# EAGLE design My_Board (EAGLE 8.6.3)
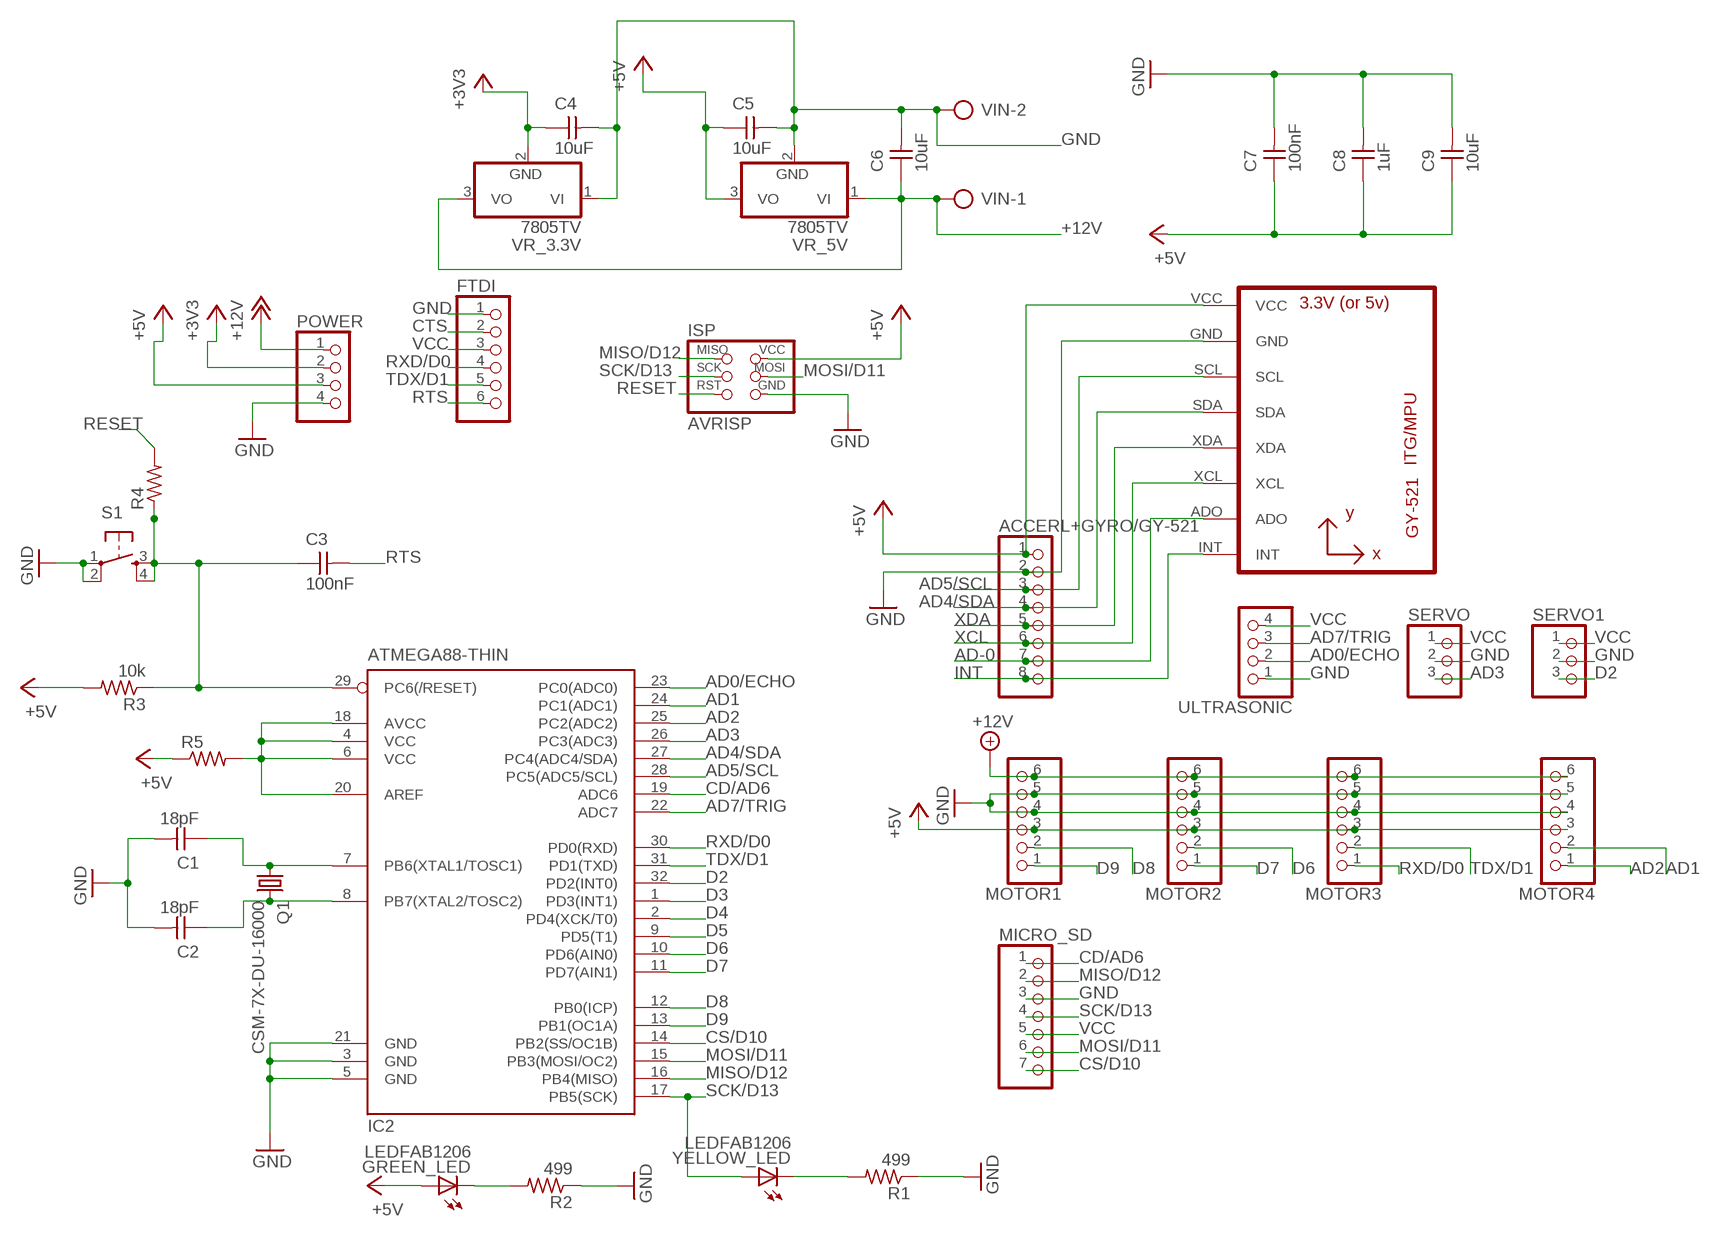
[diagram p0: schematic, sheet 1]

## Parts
ACCERL+GYRO/GY-521  PINHD-1X8  [1X08]
C1  18pF  CAP-UNPOLARIZED  [C1206]
C2  18pF  CAP-UNPOLARIZED  [C1206]
C3  100nF  CAP-UNPOLARIZEDFAB  [C1206FAB]
C4  10uF  CAP-UNPOLARIZEDFAB  [C1206FAB]
C5  10uF  CAP-UNPOLARIZEDFAB  [C1206FAB]
C6  10uF  CAP-UNPOLARIZEDFAB  [C1206FAB]
C7  100nF  CAP-UNPOLARIZEDFAB  [C1206FAB]
C8  1uF  CAP-UNPOLARIZEDFAB  [C1206FAB]
C9  10uF  CAP-UNPOLARIZEDFAB  [C1206FAB]
FTDI  PINHD-1X6  [1X06]
GREEN_LED  LEDFAB1206  [LED1206FAB]
IC2  ATMEGA88-THIN  [TQFP32-08THIN]
ISP  AVRISP  [2X03]
MICRO_SD  PINHD-1X7  [1X07]
MOTOR1  PINHD-1X6  [1X06]
MOTOR2  PINHD-1X6  [1X06]
MOTOR3  PINHD-1X6  [1X06]
MOTOR4  PINHD-1X6  [1X06]
POWER  PINHD-1X4  [1X04]
Q1  CSM-7X-DU-16000  CSM-7X-DU  [CSM-7X-DU]
R1  499  RES-US1206FAB  [R1206FAB]
R2  499  RES-US1206FAB  [R1206FAB]
R3  10k  RES-US1206FAB  [R1206FAB]
R4  RES-US1206FAB  [R1206FAB]
R5  RES-US1206FAB  [R1206FAB]
S1  6MM_SWITCH6MM_SWITCH  [6MM_SWITCH]
SERVO  PINHD-1X3  [1X03]
SERVO1  PINHD-1X3  [1X03]
U1  GY-521MPU6050  [GY-521]
ULTRASONIC  PINHD-1X4  [1X04]
VIN  AK500/2  [AK500/2]
VR_3.3V  7805TV  [TO220V]
VR_5V  7805TV  [TO220V]
YELLOW_LED  LEDFAB1206  [LED1206FAB]

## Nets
+3V3: C4.1 POWER.2 VR_3.3V.2(GND)
+12V: C6.1 MOTOR1.6 MOTOR2.6 MOTOR3.6 MOTOR4.6 POWER.1 VIN.1 VR_3.3V.3(VO) VR_5V.1(VI)
AD0/ECHO: IC2.23(PC0(ADC0)) ULTRASONIC.2
AD1: IC2.24(PC1(ADC1)) MOTOR4.2
AD2: IC2.25(PC2(ADC2)) MOTOR4.1
AD3: IC2.26(PC3(ADC3)) SERVO.3
AD4/SDA: ACCERL+GYRO/GY-521.4 IC2.27(PC4(ADC4/SDA)) U1.SDA
AD5/SCL: ACCERL+GYRO/GY-521.3 IC2.28(PC5(ADC5/SCL)) U1.SCL
AD7/TRIG: IC2.22(ADC7) ULTRASONIC.3
AD-0: ACCERL+GYRO/GY-521.7 U1.ADO
CD/AD6: IC2.19(ADC6) MICRO_SD.1
CS/D10: IC2.14(PB2(SS/OC1B)) MICRO_SD.7
CTS: FTDI.2
D2: IC2.32(PD2(INT0)) SERVO1.3
D3: IC2.1(PD3(INT1))
D4: IC2.2(PD4(XCK/T0))
D5: IC2.9(PD5(T1))
D6: IC2.10(PD6(AIN0)) MOTOR2.2
D7: IC2.11(PD7(AIN1)) MOTOR2.1
D8: IC2.12(PB0(ICP)) MOTOR1.2
D9: IC2.13(PB1(OC1A)) MOTOR1.1
GND: ACCERL+GYRO/GY-521.2 C1.2 C2.2 C4.2 C5.2 C6.2 C7.2 C8.2 C9.2 FTDI.1 IC2.3(GND) IC2.5(GND) IC2.21(GND) ISP.6(GND) MICRO_SD.3 MOTOR1.4 MOTOR1.5 MOTOR2.4 MOTOR2.5 MOTOR3.4 MOTOR3.5 MOTOR4.4 MOTOR4.5 POWER.4 R1.1 R2.1 S1.1(P) S1.2(P1) SERVO1.2 SERVO.2 U1.GND ULTRASONIC.1 VIN.2 VR_3.3V.1(VI) VR_5V.2(GND)
INT: ACCERL+GYRO/GY-521.8 U1.INT
MISO/D12: IC2.16(PB4(MISO)) ISP.1(MISO) MICRO_SD.2
MOSI/D11: IC2.15(PB3(MOSI/OC2)) ISP.4(MOSI) MICRO_SD.6
N$3: R1.2 YELLOW_LED.2(C)
N$5: C2.1 IC2.8(PB7(XTAL2/TOSC2)) Q1.2
N$6: C1.1 IC2.7(PB6(XTAL1/TOSC1)) Q1.1
N$34: GREEN_LED.2(C) R2.2
RESET: C3.1 IC2.29(PC6(/RESET)) ISP.5(RST) R3.1 R4.1 R4.2 S1.3(S) S1.4(S1)
RTS: C3.2 FTDI.6
RXD/D0: FTDI.4 IC2.30(PD0(RXD)) MOTOR3.1
SCK/D13: IC2.17(PB5(SCK)) ISP.3(SCK) MICRO_SD.4 YELLOW_LED.1(A)
TDX/D1: FTDI.5 IC2.31(PD1(TXD)) MOTOR3.2
VCC: ACCERL+GYRO/GY-521.1 C5.1 C7.1 C8.1 C9.1 FTDI.3 GREEN_LED.1(A) IC2.4(VCC) IC2.6(VCC) IC2.18(AVCC) IC2.20(AREF) ISP.2(VCC) MICRO_SD.5 MOTOR1.3 MOTOR2.3 MOTOR3.3 MOTOR4.3 POWER.3 R3.2 R5.1 R5.2 SERVO1.1 SERVO.1 U1.VCC ULTRASONIC.4 VR_5V.3(VO) ; supply symbol labelled +5V
XCL: ACCERL+GYRO/GY-521.6 U1.XCL
XDA: ACCERL+GYRO/GY-521.5 U1.XDA

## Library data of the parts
ACCERL+GYRO/GY-521 = pinhead:PINHD-1X8: PIN HEADER
C1-C9 = fab:CAP-UNPOLARIZED
FTDI MOTOR1-MOTOR4 = pinhead:PINHD-1X6: PIN HEADER
GREEN_LED YELLOW_LED = fab:LED: LED
IC2 = fab:ATMEGA88-THIN
ISP = fab:AVRISP
MICRO_SD = pinhead:PINHD-1X7: PIN HEADER
POWER ULTRASONIC = pinhead:PINHD-1X4: PIN HEADER
Q1 = crystal:CSM-7X-DU: SMD CRYSTAL; OC_FARNELL: unknown; OC_NEWARK: unknown
R1-R5 = fab:RES-US: Resistor (US Symbol)
S1 = fab:6MM_SWITCH: OMRON SWITCH
SERVO SERVO1 = pinhead:PINHD-1X3: PIN HEADER
U1 = gy-521:GY-521
VIN = con-ptr500:AK500/2: CONNECTOR; OC_FARNELL: unknown; OC_NEWARK: unknown
VR_3.3V VR_5V = linear:78*: Positive VOLTAGE REGULATOR Source: http://cache.national.com/ds/LM/LM78L05.pdf http://www.fairchildsemi.com/ds/LM/LM7805.pdf

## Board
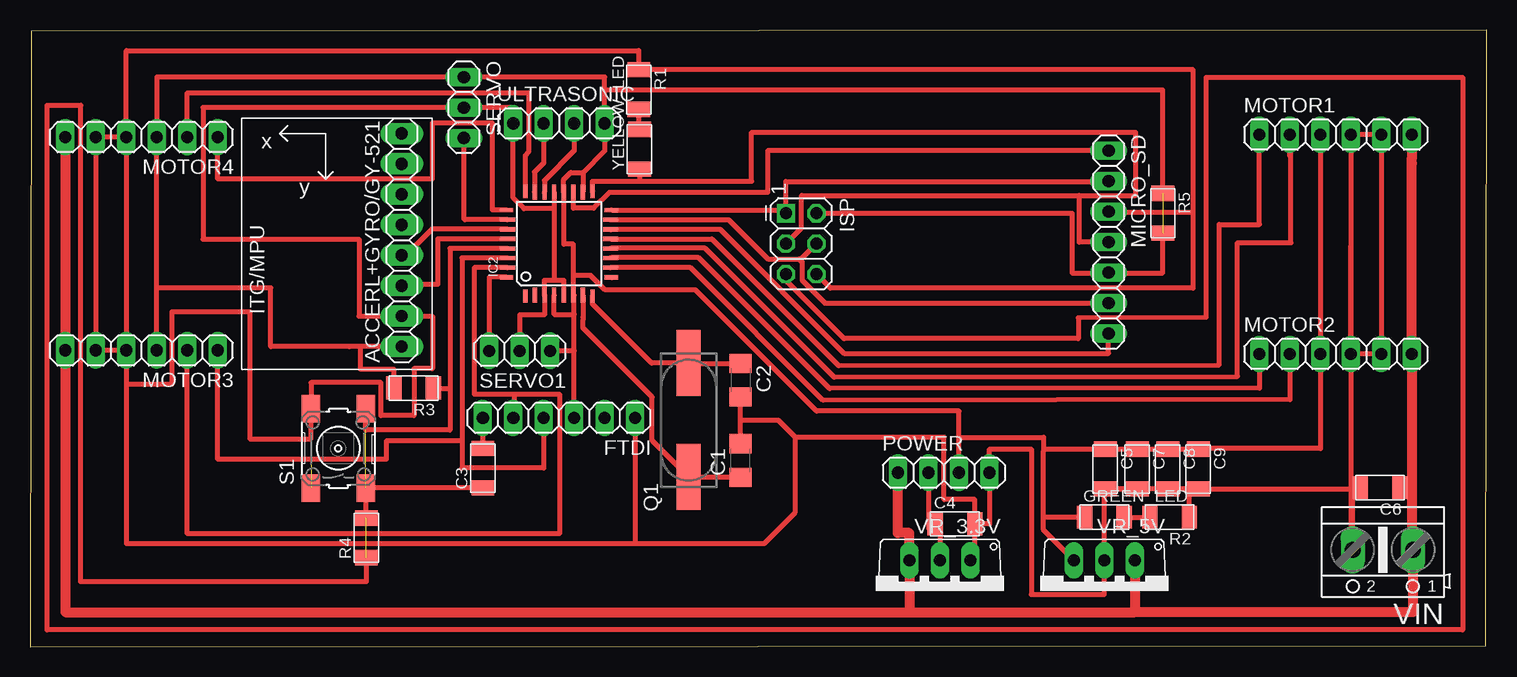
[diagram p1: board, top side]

Size 121.44 x 51.45 mm. Coordinates in mm from the lower left corner, seen from the top.
Outline: 0,0 121.34,0.1 121.44,51.45 0.1,51.35 0,0
Copper layers (1*16): Top 0.035mm / dielectric 1.5mm / Bottom 0.035mm
Design rules "default": minimum track width 6mil, minimum drill 0.35mm, track to track 6mil, track to pad 6mil, pad to pad 6mil, via to via 6mil, smd to smd 6mil, copper to edge 40mil, drill to drill 6mil, minimum pad ring 10mil, minimum via ring 8mil, stop-mask expansion 4mil, vias tented up to drill 0mil, thermal gap 10mil

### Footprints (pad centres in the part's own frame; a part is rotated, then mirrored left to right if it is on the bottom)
1X08 = drill 1.016 long: 1 -8.89,0; 2 -6.35,0; 3 -3.81,0; 4 -1.27,0; 5 1.27,0; 6 3.81,0; 7 6.35,0; 8 8.89,0
C1206 = smd 1.6 x 1.8: 1 -1.4,0; 2 1.4,0
C1206FAB = smd 1.27 x 1.905: 1 -1.651,0; 2 1.651,0
1X06 = drill 1.016 long: 1 -6.35,0; 2 -3.81,0; 3 -1.27,0; 4 1.27,0; 5 3.81,0; 6 6.35,0
LED1206FAB = smd 1.27 x 1.905: 1 -1.651,0; 2 1.651,0
TQFP32-08THIN = smd 1.118 x 0.356: 1 -4.369,2.8; 8 -4.369,-2.8; 17 4.369,-2.8; 24 4.369,2.8 | smd 1.27 x 0.356: 2 -4.293,2; 3 -4.293,1.2; 4 -4.293,0.4; 5 -4.293,-0.4; 6 -4.293,-1.2; 7 -4.293,-2; 18 4.293,-2; 19 4.293,-1.2; 20 4.293,-0.4; 21 4.293,0.4; 22 4.293,1.2; 23 4.293,2 | smd 0.356 x 1.118: 9 -2.8,-4.369; 16 2.8,-4.369; 25 2.8,4.369; 32 -2.8,4.369 | smd 0.356 x 1.27: 10 -2,-4.293; 14 1.2,-4.293; 15 2,-4.293; 26 2,4.293; 27 1.2,4.293; 31 -2,4.293 | smd 0.35 x 1.27: 11 -1.2,-4.293; 12 -0.4,-4.293; 13 0.4,-4.293; 28 0.4,4.293; 29 -0.4,4.293; 30 -1.2,4.293
2X03 = drill 1.016 square: 1 -2.54,-1.27 | drill 1.016 octagon: 2 -2.54,1.27; 3 0,-1.27; 4 0,1.27; 5 2.54,-1.27; 6 2.54,1.27
1X07 = drill 1.016 long: 1 -7.62,0; 2 -5.08,0; 3 -2.54,0; 4 0,0; 5 2.54,0; 6 5.08,0; 7 7.62,0
1X04 = drill 1.016 long: 1 -3.81,0; 2 -1.27,0; 3 1.27,0; 4 3.81,0
CSM-7X-DU = smd 5.5 x 2: 1 -4.75,0; 2 4.75,0
R1206FAB = smd 1.27 x 1.905: 1 -1.651,0; 2 1.651,0
6MM_SWITCH = smd 2.286 x 1.524: 1 -3.302,2.286; 2 3.302,2.286; 3 -3.302,-2.286; 4 3.302,-2.286
1X03 = drill 1.016 long: 1 -2.54,0; 2 0,0; 3 2.54,0
GY-521 = drill 0.8 pad 1.778 long: ADO -8.89,-6.35; GND -8.89,6.35; INT -8.89,-8.89; SCL -8.89,3.81; SDA -8.89,1.27; VCC -8.89,8.89; XCL -8.89,-3.81; XDA -8.89,-1.27
AK500/2 = drill 1.321 long: 1 -2.515,0; 2 2.515,0
TO220V = drill 1.016 long: 1 -2.54,-2.54; 2 0,-2.54; 3 2.54,-2.54

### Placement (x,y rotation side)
ACCERL+GYRO/GY-521  30.99,33.93 90 top
C1  59.23,15.54 90 top
C2  59.23,22.25 270 top
C3  37.74,14.91 90 top
C4  77.11,10.26 0 top
C5  89.64,14.83 270 top
C6  112.55,13.28 180 top
C7  92.3,14.83 270 top
C8  94.84,14.83 270 top
C9  97.38,14.83 270 top
FTDI  44.09,19.1 180 top
GREEN_LED  89.56,10.82 0 top
IC2  44.09,33.63 90 top
ISP  64.29,33.63 270 top
MICRO_SD  89.92,33.76 270 top
MOTOR1  108.84,42.72 0 top
MOTOR2  108.84,24.43 0 top
MOTOR3  9.3,24.74 180 top
MOTOR4  9.3,42.52 180 top
POWER  76.17,14.53 0 top
Q1  54.91,18.92 90 top
R1  50.75,46.48 270 top
R2  95,10.82 180 top
R3  31.98,21.59 180 top
R4  28.04,9.09 90 top
R5  94.44,36.17 270 top
S1  25.7,16.56 90 top
SERVO  36.17,44.98 270 top
SERVO1  40.82,24.69 180 top
U1  22.1,33.93 180 top
ULTRASONIC  44.09,43.66 0 top
VIN  112.78,8.1 180 top
VR_3.3V  75.84,4.67 180 top
VR_5V  89.56,4.67 180 top
YELLOW_LED  50.8,41.5 90 top

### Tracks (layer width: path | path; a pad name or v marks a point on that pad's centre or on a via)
+3V3
  Top 0.406: 75.84,9.86 75.84,10.01 75.59,10.26 C4.1 | 75.84,9.86 VR_3.3V.2 | POWER.2 74.9,9.86 75.84,9.86
+12V
  Top 0.406: C6.1 115.11,13.28 115.19,13.36
  Top 0.813: MOTOR4.6 MOTOR3.6 2.95,2.9 73.3,2.9 | 73.3,2.9 VR_3.3V.3 73.3,9.5 72.34,9.5 72.34,14.53 POWER.1 | 73.3,2.9 92.1,2.9 | VR_5V.1 92.1,2.9 | 92.1,2.9 115.29,2.9 VIN.1 115.19,8.1 115.19,13.36 MOTOR2.6 115.19,40.34 115.19,40.79 MOTOR1.6
AD0/ECHO
  Top 0.406: IC2.23 42.06,37.95 42.06,39.6 42.82,40.36 ULTRASONIC.2
AD1
  Top 0.406: IC2.24 41.29,40.99 41.55,41.25 41.55,46.2 13.11,46.2 MOTOR4.2
AD2
  Top 0.406: IC2.25 38.56,36.43 38.56,43.69 33.53,43.69 33.53,39.01 15.65,39.01 MOTOR4.1
AD3
  Top 0.406: IC2.26 36.25,35.63 36.17,35.71 SERVO.3
AD4/SDA
  Top 0.406: 30.99,32.61 U1.SDA 31.95,32.66 31.95,33.27 33.51,34.83 IC2.27
AD5/SCL
  Top 0.406: IC2.28 33.99,34.03 33.99,30.23 30.99,30.23 U1.SCL
AD7/TRIG
  Top 0.406: ULTRASONIC.3 45.36,41.38 42.89,38.91 IC2.22
CD/AD6
  Top 0.406: IC2.19 45.29,36.58 46.99,36.58 48.31,37.9 61.49,37.9 61.49,41.38 MICRO_SD.1
CS/D10
  Top 0.406: 48.42,34.8 IC2.14 57.53,34.83 67.87,24.49 89.92,24.49 MICRO_SD.7
D2
  Top 0.406: SERVO1.3 38.28,30.83 IC2.32
D5
  Top 0.406: 48.51,30.79 IC2.9
D6
  Top 0.406: MOTOR2.2 105.03,20.62 66.12,20.57 55.06,31.63 IC2.10
D7
  Top 0.406: IC2.11 48.42,32.46 55.73,32.46 66.65,21.54 102.49,21.59 MOTOR2.1
D8
  Top 0.406: 105.03,42.34 105.03,40.92 105.05,40.92 | 105.03,42.34 MOTOR1.2 | IC2.12 48.42,33.25 56.29,33.25 67.03,22.5 100.66,22.55 100.66,33.71 105.11,33.71 105.11,42.34 105.03,42.34
D9
  Top 0.406: IC2.13 56.85,34.03 67.41,23.47 99.14,23.52 99.14,35.23 102.49,35.23 MOTOR1.1
GND  (1 unrouted)
  Top 0.406: MOTOR2.4 MOTOR1.4 MOTOR1.5 MOTOR2.5 MOTOR2.4 | MOTOR2.4 110.11,33.45 | C9.2 C8.2 | C8.2 C7.2 | C9.2 96.65,13.18 R2.1 | C8.2 92.35,13.18 | 78.71,10.77 78.71,10.26 | 78.71,10.26 78.71,7.54 VR_3.3V.1 | 42.93,29.3 IC2.3 | IC2.3 42.89,30.58 43.69,30.58 | IC2.5 44.49,30.58 43.69,30.58 | MOTOR4.4 MOTOR4.5 MOTOR3.5 MOTOR3.4 | C4.2 78.71,10.26 | 89.56,13.13 89.92,13.14 | 89.92,13.14 C7.2 | C7.2 C5.2 | C6.2 110.26,13.28 VIN.2 110.11,8.1 110.11,13.18 | 97.38,13.23 C9.2 | 89.92,13.14 89.56,13.14 VR_5V.2 89.56,4.37 83.46,4.37 83.46,16.51 79.98,16.51 POWER.4 79.98,10.26 C4.2 | 43.69,30.58 IC2.21 43.69,36.57 43.71,36.55 41.17,36.55 40.28,37.44 ULTRASONIC.1 40.28,44.98 SERVO.2 14.43,44.98 14.43,34.01 27.43,34.01 27.43,27.58 U1.GND 33.55,27.58 33.55,23.22 32,23.22 32,19.3 29.26,19.3 29.26,22.05 23.42,22.05 S1.2 23.42,19.61 23.42,17.35 18.31,17.35 18.31,27.97 11.84,27.97 11.84,21.92 8.03,21.92 MOTOR3.4 | C1.2 59.23,19 | 59.23,19 C2.2 | 63.81,17.48 62.38,18.9 59.33,18.9 59.23,19 | 63.81,17.48 63.81,11.23 61.21,8.64 50.44,8.64 | MOTOR4.4 MOTOR3.4 | MOTOR4.4 8.03,49.73 50.75,49.73 R1.1 96.98,48.13 96.98,36.22 | MOTOR2.4 110.11,13.18 | 89.92,36.32 MICRO_SD.3 89.92,36.22 96.98,36.22 | C4.2 78.77,12.29 76.2,12.29 76.2,17.48 63.81,17.48 | IC2.3 42.89,27.69 40.82,27.69 SERVO1.2 | MOTOR3.4 8.03,20.93 8.03,8.64 18.39,8.64 50.44,8.64 | ISP.6 66.73,29.92 96.98,29.92 96.98,36.22 | FTDI.1 50.44,8.64 | C9.2 110.11,13.18
MISO/D12
  Top 0.406: IC2.16 62.76,36.43 ISP.1 63.02,38.81 89.92,38.81 MICRO_SD.2
MOSI/D11
  Top 0.406: 89.28,28.68 MICRO_SD.6 66.27,28.68 64.36,30.58 64.36,32.11 64.11,32.36 | IC2.15 58.25,35.63 61.52,32.36 64.11,32.36 | ISP.4 64.29,32.36 64.11,32.36
N$3
  Top 0.406: YELLOW_LED.2 R1.2
N$5
  Top 0.406: C2.1 54.94,23.65 Q1.2 51.82,23.67 46.89,28.6 IC2.8
N$6
  Top 0.406: 46.08,29.34 IC2.7 46.09,27.48 46.09,27.26 46.09,26.6 51.87,20.83 51.87,17.22 Q1.1 59.23,14.17 C1.1
N$34
  Top 0.406: GREEN_LED.2 R2.2
RESET  (2 unrouted)
  Top 0.406: IC2.29 35,33.23 35,21.54 | S1.4 27.99,18.09 35,18.09 35,21.54 | C3.1 S1.3 28.04,13.26 R4.2 | ISP.5 63.02,30.56 67.87,25.7 87.38,25.7 87.38,27.43 98.04,27.48 98.04,47.5 119.43,47.5 119.43,1.42 1.42,1.42 1.42,45.16 4.22,45.16 | 4.27,45.16 4.22,45.16 | R3.1 33.63,21.54 35,21.54 | 4.22,45.16 4.22,5.44 28.04,5.44 R4.1
RTS
  Top 0.406: FTDI.6 C3.2
RXD/D0
  Top 0.406: IC2.30 36.02,32.43 36.02,17.17 | 36.02,17.17 36.02,14.91 42.82,14.91 FTDI.4 | 36.02,17.17 29.69,17.17 29.69,15.65 15.65,15.65 MOTOR3.1
SCK/D13
  Top 0.406: 46.89,38.08 IC2.17 | IC2.17 | IC2.17 46.89,38.83 46.89,38.84 50.85,38.84 | ISP.3 64.29,34.9 64.31,34.9 64.31,37.64 87.48,37.64 | MICRO_SD.4 87.48,33.76 87.48,37.64 | 87.48,37.64 92.15,37.64 92.15,42.93 60.15,42.93 60.15,38.84 50.85,38.84 | 50.85,38.84 50.85,39.85 YELLOW_LED.1
TDX/D1
  Top 0.406: IC2.31 37.03,31.63 37.03,21.08 40.34,21.08 | 40.34,21.08 40.34,19.1 FTDI.5 | 40.34,21.08 44.15,21.08 44.15,9.45 13.11,9.45 MOTOR3.2
VCC  (1 unrouted)
  Top 0.406: 46.09,39.57 47.9,41.38 ULTRASONIC.4 47.9,46.43 | 46.09,39.57 IC2.18 | 46.09,39.57 45.08,39.57 44.49,38.98 IC2.20 44.5,33.58 45.29,33.58 45.29,30.99 | VR_5V.3 84.48,9.75 84.48,10.82 | 84.48,10.82 84.48,16.36 | MOTOR1.3 MOTOR2.3 107.57,16.55 97.45,16.55 | 97.51,16.61 97.45,16.55 | 97.45,16.55 C9.1 C8.1 C7.1 C5.1 84.48,16.48 | 84.61,16.48 84.48,16.36 | 84.48,16.48 84.48,17.48 77.44,17.48 POWER.3 77.44,19.66 65.58,19.66 55.47,29.77 47.96,29.77 46.74,30.99 45.29,30.99 | 84.48,16.48 84.48,16.36 | GREEN_LED.1 84.48,10.82 | 45.29,30.99 IC2.6 45.36,29.34 45.36,27.74 | MOTOR3.3 10.57,29.95 | 10.57,29.95 MOTOR4.3 10.57,47.52 SERVO.1 47.9,47.52 47.9,46.43 | 45.36,24.69 45.36,27.74 | U1.VCC 27.53,25.04 | 27.53,25.04 26.62,25.04 20.07,25.04 20.07,29.95 10.97,29.95 10.57,29.95 | IC2.4 43.69,27.74 45.36,27.74 | ISP.2 86.87,36.17 86.87,31.19 89.92,31.19 | 89.92,31.19 MICRO_SD.5 | 45.36,24.69 SERVO1.1 | R5.2 94.44,31.19 89.92,31.19 | R5.1 94.44,46.43 47.9,46.43 | FTDI.3 45.36,24.69 | 27.53,25.04 27.53,23.16 30.33,23.16 R3.2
